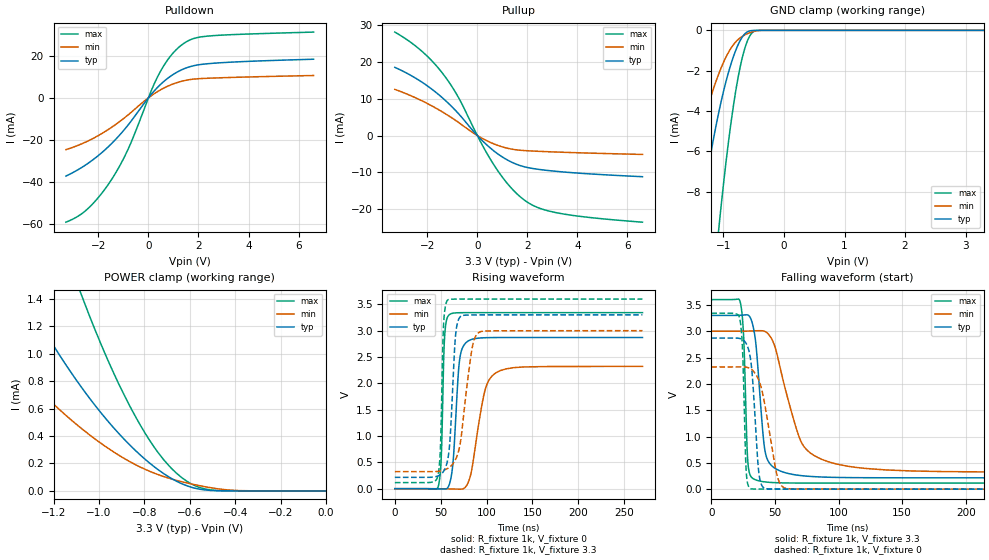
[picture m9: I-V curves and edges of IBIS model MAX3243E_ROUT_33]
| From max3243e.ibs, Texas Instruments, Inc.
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[Model]   MAX3243E_ROUT_33
Model_type  3-state
Enable   Active-High
Vref =   0
Rref =   3000
Cref =   150p
Vmeas =   1.5
| variable   typ   min   max
C_comp   3.23pF   2.85pF   3.42pF
| C_pullup   3.88pF   3.10pF   5.05pF
| C_pulldown   4.16pF   3.17pF   5.48pF
| C_tri-state   3.23pF   2.85pF   3.42pF
[Temperature Range]   40   100   -40
| Ambient temperature   25   85   -40
[Voltage range]   3.3   3   3.6
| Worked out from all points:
|   slope of the pulldown table from 0 to 0.495 V, typ, clamps not added: 75.9 ohm
|   slope of the pullup table from 0 to 0.495 V, typ, clamps not added: 152 ohm
|   GND clamp passes 1 mA (typ) near -0.80 V on its own axis
|   POWER clamp passes 1 mA (typ) near -1.18 V on its own axis
|   rising waveform, R_fixture 1k, V_fixture 0: 20-80 % time 5.91ns typ, 13.3ns min, 2.92ns max; typ from 0 V to 2.87 V
|   falling waveform, R_fixture 1k, V_fixture 3.3: 20-80 % time 6.22ns typ, 18.9ns min, 2.67ns max; typ from 3.3 V to 0.215 V
|   rising waveform, R_fixture 1k, V_fixture 3.3: 20-80 % time 5.53ns typ, 11.2ns min, 2.85ns max; typ from 0.215 V to 3.3 V
|   falling waveform, R_fixture 1k, V_fixture 0: 20-80 % time 4.69ns typ, 10ns min, 2.36ns max; typ from 2.87 V to 0 V
[GND Clamp]
| MAX3243E_ROUT_33
|   Voltage   I(typ)   I(min)   I(max)
-3.3V     -76.07mA   -49.44mA   -130.6mA
-1.69V    -16.48mA   -9.519mA   -34.03mA
-1.395V   -9.606mA   -5.345mA   -21.06mA
-1.25V    -6.826mA   -3.717mA   -15.54mA
-1.095V   -4.324mA   -2.298mA   -10.39mA
-1.065V   -3.899mA   -2.062mA   -9.489mA
-930mV    -2.228mA   -1.167mA   -5.852mA
-805mV    -1.056mA   -599.8uA   -3.16mA
-710mV    -434.7uA   -343.6uA   -1.633mA
-605mV    -76.59uA   -167.5uA   -533.3uA
-425mV    -293.2nA   -12.5uA    -3.703uA
3.3V      6.8pA      192.8nA    6.312pA
[POWER Clamp]
| MAX3243E_ROUT_33
|   Voltage   I(typ)   I(min)   I(max)
-3.3V     11.5mA     7.221mA    19.78mA
-1.625V   2.417mA    1.44mA     4.558mA
-1.6V     2.324mA    1.385mA    4.387mA
-1.335V   1.438mA    856.2uA    2.732mA
-1.315V   1.378mA    821.1uA    2.619mA
-1.08V    761.5uA    458.7uA    1.44mA
-935mV    459.3uA    283.6uA    857.8uA
-835mV    287.8uA    187.8uA    529uA
-740mV    155.5uA    119.2uA    280.4uA
-635mV    52.23uA    66.96uA    96.54uA
-510mV    3.805uA    24.04uA    7.633uA
-48.03fV  6.8pA      37.29pA    7.219pA
[Pulldown]
| MAX3243E_ROUT_33
|   Voltage   I(typ)   I(min)   I(max)
-3.3V     -37.36mA   -24.73mA   -59.37mA
-2.41V    -31.22mA   -20.56mA   -52.77mA
-1.945V   -26.98mA   -17.62mA   -46.74mA
-1.49V    -22.02mA   -14.21mA   -39.27mA
-785mV    -12.55mA   -7.874mA   -23.77mA
105mV     1.553mA    924uA      3.189mA
405mV     5.483mA    3.267mA    10.97mA
845mV     9.985mA    5.942mA    19.36mA
1.325V    13.36mA    7.893mA    25.21mA
1.77V     15.21mA    8.872mA    28.15mA
2.345V    16.25mA    9.321mA    29.43mA
6.6V      18.42mA    10.64mA    31.37mA
[Pullup]
| MAX3243E_ROUT_33
|   Voltage   I(typ)   I(min)   I(max)
-3.3V     18.59mA    12.59mA    28.19mA
-2.245V   14.68mA    9.565mA    23.13mA
-1.79V    12.48mA    7.972mA    20.15mA
-1.375V   10.15mA    6.348mA    16.82mA
-755mV    5.974mA    3.589mA    10.36mA
130mV     -924.9uA   -518.6uA   -1.72mA
660mV     -4.185mA   -2.269mA   -7.977mA
1.255V    -6.853mA   -3.532mA   -13.52mA
1.84V     -8.438mA   -4.072mA   -17.38mA
2.415V    -9.176mA   -4.283mA   -19.61mA
3.215V    -9.787mA   -4.504mA   -21.09mA
6.6V      -11.21mA   -5.144mA   -23.6mA
[Ramp]
| MAX3243E_ROUT_33
| variable   typ   min   max
dV/dt_r   1.73/5.92E-09   1.40/1.33E-08   2.01/2.92E-09
dV/dt_f   1.86/6.24E-09   1.61/1.89E-08   2.10/2.69E-09
R_load = 1k
[Rising Waveform]
| MAX3243E_ROUT_33
R_fixture =   1k
C_fixture =   0
L_fixture =   0
V_fixture =   0
V_fixture_min = 0
V_fixture_max = 0
|   Time   V(typ)   V(min)   V(max)
0s        331.6pV    2.084nV    131.1pV
47.4ns    -2.916mV   -917.8uV   45.8mV
50.7ns    -5.103mV   -1.554mV   636.3mV
54.3ns    -7.604mV   -2.351mV   2.891V
59.7ns    95.84mV    -4.286mV   3.307V
70.5ns    2.429V     -9.061mV   3.341V
78.8ns    2.79V      75.58mV    3.342V
98ns      2.866V     1.849V     3.342V
109.8ns   2.869V     2.195V     3.342V
269.9ns   2.87V      2.321V     3.342V
[Falling Waveform]
| MAX3243E_ROUT_33
R_fixture =   1k
C_fixture =   0
L_fixture =   0
V_fixture =   3.3
V_fixture_min = 3
V_fixture_max = 3.6
|   Time   V(typ)   V(min)   V(max)
0s        3.3V       3V         3.6V
22.8ns    3.303V     3V         3.548V
25.4ns    3.308V     3V         2.903V
28.7ns    3.308V     3.002V     525.4mV
33.5ns    3.019V     3.007V     191.7mV
42.1ns    742.7mV    2.995V     138.1mV
52.3ns    365.6mV    2.501V     121.9mV
70ns      259mV      934mV      116.1mV
87ns      230.7mV    565mV      115.3mV
269.9ns   215.4mV    324.6mV    115.2mV
[Rising Waveform]
| MAX3243E_ROUT_33
R_fixture =   1k
C_fixture =   0
L_fixture =   0
V_fixture =   3.3
V_fixture_min = 3
V_fixture_max = 3.6
|   Time   V(typ)   V(min)   V(max)
0s        215.4mV    323.9mV    115.2mV
46.6ns    239.6mV    328.4mV    221.9mV
49.8ns    267.8mV    336.6mV    818.1mV
53.2ns    331.7mV    351.4mV    3.129V
57.6ns    546.3mV    384.2mV    3.582V
66.2ns    2.909V     555.9mV    3.599V
72.1ns    3.277V     951.5mV    3.6V
83.9ns    3.298V     2.632V     3.6V
91.9ns    3.299V     2.969V     3.6V
269.9ns   3.3V       3V         3.6V
[Falling Waveform]
| MAX3243E_ROUT_33
R_fixture =   1k
C_fixture =   0
L_fixture =   0
V_fixture =   0
V_fixture_min = 0
V_fixture_max = 0
|   Time   V(typ)   V(min)   V(max)
0s        2.87V      2.321V     3.342V
22.4ns    2.862V     2.322V     3.234V
24.6ns    2.842V     2.322V     2.616V
27.4ns    2.767V     2.317V     355.7mV
30.7ns    2.49V      2.29V      11.67mV
37.2ns    346.9mV    2.076V     1.883mV
41.9ns    16.42mV    1.627V     1.109mV
51.5ns    2.65mV     282.4mV    379.5uV
58.2ns    1.739mV    17.74mV    179.4uV
269.9ns   6.095nV    5.102uV    121.3pV
